TYPE dut_GB_Output :
STRUCT
								    									
	Q200_00			:BOOL;	//	OX_Pump_On
	Q200_01			:BOOL;	//	Spare1
	Q200_02			:BOOL;	//	Spare2
	Q200_03			:BOOL;	//	Spare3
	Q200_04			:BOOL;	//	Spare4
	Q200_05			:BOOL;	//	Spare5
	Q200_06			:BOOL;	//	Spare6
	Q200_07			:BOOL;	//	Spare7
	Q200_08			:BOOL;	//	Spare8
	Q200_09			:BOOL;	//	Spare9
	Q200_10			:BOOL;	//	Spare10
	Q200_11			:BOOL;	//	Spare11
	Q200_12			:BOOL;	//	Spare12
	Q200_13			:BOOL;	//	Spare13
	Q200_14			:BOOL;	//	Spare14
	Q200_15			:BOOL;	//	Spare15
	
	QEV				:ARRAY[1..5]OF dut_EX260_SEC;	//阀岛输出
	
END_STRUCT
END_TYPE
